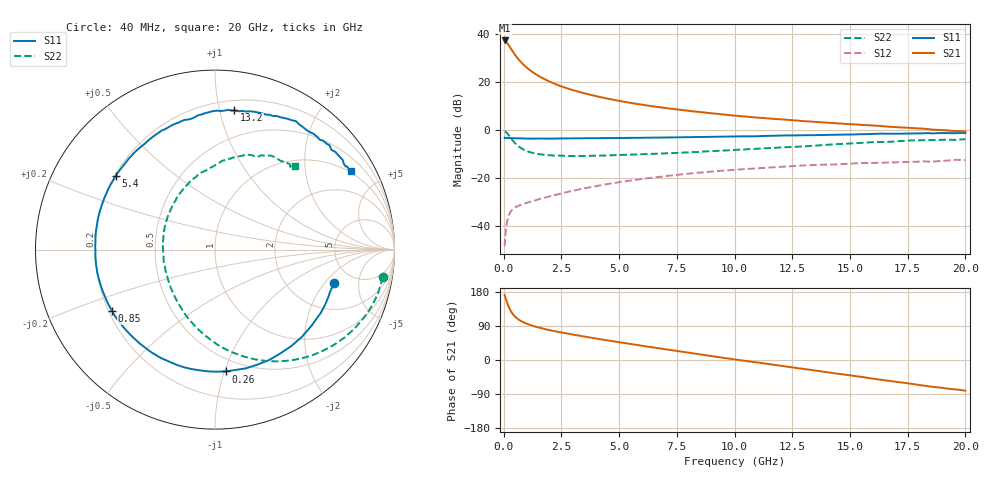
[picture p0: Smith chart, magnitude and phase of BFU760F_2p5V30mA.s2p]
! Filename:  P:\Prog\Test\Noise\ATS_data\Testdata_Net\Split files Spar\BFU760F_2W_C1_Bias7_2.5V_5mA_30mA_D.s2p
! Date/Time: Mon 06/Feb/2012 15:08:28
! BFU760_2W_C1_Bias7_2.5V_5mA_30mA_R.s2p
! MDIF S-parameter v. bias file
! BFU760_2W_C1_2.5V_5mA_30mA
! Date/time Fri Mar 18 11:16:19 2011
! VAR V_out= 2.5000
! VAR I_out= 29.9650
! VAR V_in= 0.7879
! VAR I_in= 0.0989
! Device data file deembeded for feedlines and parallel
! Original file: \Split files Spar\BFU760_2W_C1_Bias7_2.5V_5mA_30mA_R.s2p
! Feed-files: PR003V01_101208_Feed1.s2p, PR003V01_101208_Feed2.s2p
! Parallel-file: PR003V01_101208_Par.s2p
# MHz S MA R 50
!  Freq-MHz  S11-mag  S11-arg  S21-mag  S21-arg  S12-mag  S12-arg  S22-mag  S22-arg
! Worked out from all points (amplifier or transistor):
!   167 points, 40 MHz to 20 GHz, reference 50 ohm
!   highest |S21| = 37.3 dB at 40 MHz (marker M1)
!   |S21| within 3 dB of that: start of sweep to 286.4 MHz
!   unconditionally stable (mu >= 1): 3.703 GHz to 13.82 GHz
!   at 550 MHz: K = 0.35, MSG = 31.2 dB, |S12| = -31.9 dB
!   at 4.2 GHz: K = 1.02, MAG = 17.5 dB, |S12| = -22.9 dB
!   at 20 GHz: K = 0.91, MSG = 5.9 dB, |S12| = -12.4 dB
!   S11 on the Smith chart (normalised r, x): 40 MHz: 3.56, -2.54; 260 MHz: 0.40, -1.01; 850 MHz: 0.21, -0.26; 5.4 GHz: 0.20, +0.32; 13.2 GHz: 0.28, +1.11; 20 GHz: 0.96, +3.49
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40  0.691 -15.6  73.38 171.5  0.003842 72.4  0.9471 -9.3
50  0.6829 -19.8  73 168.9  0.004579 67.4  0.9432 -12.2
90  0.684 -34.8  70.56 161.2  0.008092 70.2  0.9204 -22.2
140  0.6853 -51.8  66.24 152.1  0.0119 65.1  0.873 -34.1
200  0.6829 -69.9  60.2 142.6  0.01563 58.7  0.8049 -46.5
260  0.6813 -85.0  54.39 134.6  0.01845 53.7  0.7356 -57.4
300  0.6795 -93.7  50.66 130.0  0.01998 50.7  0.6932 -63.8
380  0.6766 -108.2  44.22 122.4  0.02229 46.5  0.6165 -74.9
500  0.6719 -123.6  36.37 114.1  0.02473 42.4  0.5304 -88.5
650  0.6687 -136.9  29.38 106.6  0.02681 40.1  0.4553 -101.6
850  0.6683 -149.1  23.19 99.6  0.02904 39.2  0.3949 -115.3
1250  0.6674 -163.8  16.14 90.3  0.03334 40.3  0.3359 -134.4
1800  0.6676 -175.9  11.3 81.3  0.03957 42.6  0.3045 -151.8
2450  0.6693 174.5  8.29 73.2  0.04744 44.3  0.2934 -165.8
3400  0.6752 163.1  5.996 62.9  0.06016 43.9  0.2904 179.5
5400  0.6886 143.6  3.757 43.0  0.08801 37.7  0.3056 156.2
6800  0.6999 131.6  2.97 30.1  0.1072 31.1  0.3247 142.8
10200  0.7405 104.5  1.965 -0.1  0.1515 11.5  0.3923 113.8
13200  0.7835 82.1  1.516 -25.3  0.1863 -7.7  0.4652 90.8
13400  0.7816 80.4  1.492 -27.0  0.1877 -9.5  0.4728 89.5
16800  0.8404 54.6  1.165 -55.8  0.212 -31.4  0.5734 64.8
20000  0.8718 30.0  0.9416 -81.1  0.2393 -53.1  0.6448 46.3
